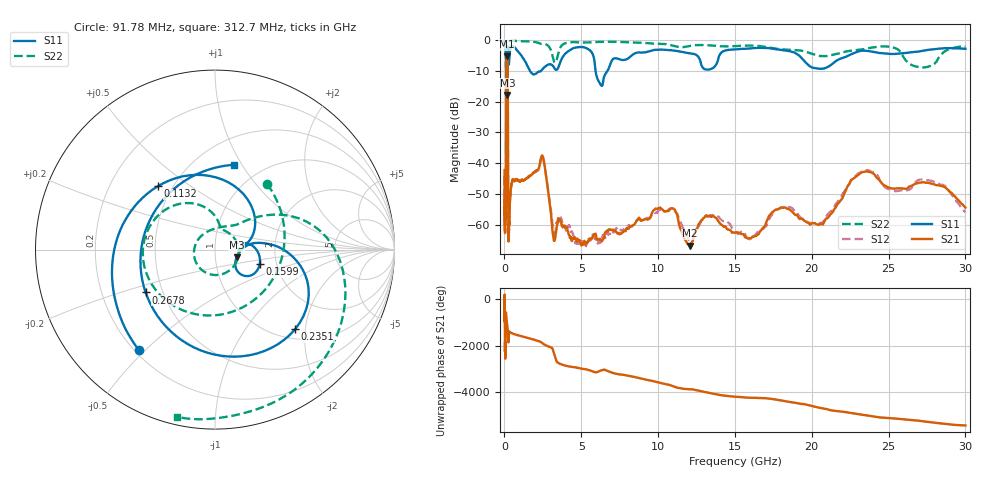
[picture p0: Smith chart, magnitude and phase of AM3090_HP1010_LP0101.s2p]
! Date/Time: Thu, Feb 28, 2019 2:04 PM
! Network Analyzer: Agilent Technologies E8364B Rev: A.07.50.67
! Sweep from 0.010 to 30.000 GHz, 1601 Points, Sweep Type: LOG
! Power Supply: 5.023 V, 0.002 A
# Hz S DB R 50
!freq MagS11 AngS11 MagS21 AngS21 MagS12 AngS12 MagS22 AngS22
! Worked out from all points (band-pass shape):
!   1601 points, 10 MHz to 30 GHz, reference 50 ohm
!   highest |S21| = -5.26 dB at 161.5 MHz (marker M1); lowest = -66.8 dB at 12.07 GHz (marker M2)
!   |S21| within 3 dB of the highest: 127.1 MHz to 205.2 MHz (78.12 MHz wide, 47 % of centre)
!   lowest |S11| = -17.8 dB at 192.5 MHz (marker M3), VSWR 1.29, Z = 63.4 - j5.61 ohm
!   |S11| at or under -10 dB: 123 MHz to 212.9 MHz (89.88 MHz wide, 53.5 % of centre); 1.656 GHz to 2.381 GHz (725.2 MHz wide, 35.9 % of centre); 5.927 GHz to 6.709 GHz (782.4 MHz wide, 12.4 % of centre)
!   |S22| runs from -19.4 to -0.1 dB; largest |S21 - S12| = 0.013
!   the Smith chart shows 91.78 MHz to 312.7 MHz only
!   S11 on the Smith chart (normalised r, x): 91.78 MHz: 0.22, -0.48; 113.2 MHz: 0.42, +0.38; 159.9 MHz: 1.63, -0.29; 235.1 MHz: 1.20, -1.76; 267.8 MHz: 0.40, -0.24; 312.7 MHz: 0.75, +0.93
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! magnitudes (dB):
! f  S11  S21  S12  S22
! 10 MHz  -0.3  -42.3  -44.4  -0.5
! 38.04 MHz  -0.5  -61.4  -59.7  -1.3
! 91.78 MHz  -3.1  -52.3  -52.1  -6.6
! 113.2 MHz  -6.5  -20.8  -20.8  -7.9
! 144.7 MHz  -14.1  -5.5  -5.5  -18.3
! 159.9 MHz  -11.6  -5.3  -5.2  -17.1
! 161.5 MHz  -11.6  -5.3  -5.2  -17.0
! 192.5 MHz  -17.8  -6.3  -6.3  -19.1
! 214.9 MHz  -9.3  -12.8  -12.7  -11.5
! 235.1 MHz  -4.0  -40.0  -39.6  -2.7
! 267.8 MHz  -6.9  -65.0  -64.7  -0.8
! 312.7 MHz  -6.3  -60.0  -58.9  -0.4
! 550.5 MHz  -2.0  -45.4  -45.4  -0.2
! 2.084 GHz  -10.8  -42.4  -42.6  -0.7
! 2.533 GHz  -9.1  -38.6  -38.4  -1.3
! 3.236 GHz  -9.0  -65.2  -62.6  -7.1
! 7.926 GHz  -6.3  -61.3  -61.7  -0.7
! 10.65 GHz  -3.3  -55.6  -55.2  -1.5
! 12.07 GHz  -4.3  -66.8  -65.0  -2.0
! 20.31 GHz  -9.2  -59.9  -59.8  -4.9
! 23.48 GHz  -3.5  -42.8  -42.4  -2.9
! 30 GHz  -2.8  -54.5  -56.0  -2.1
